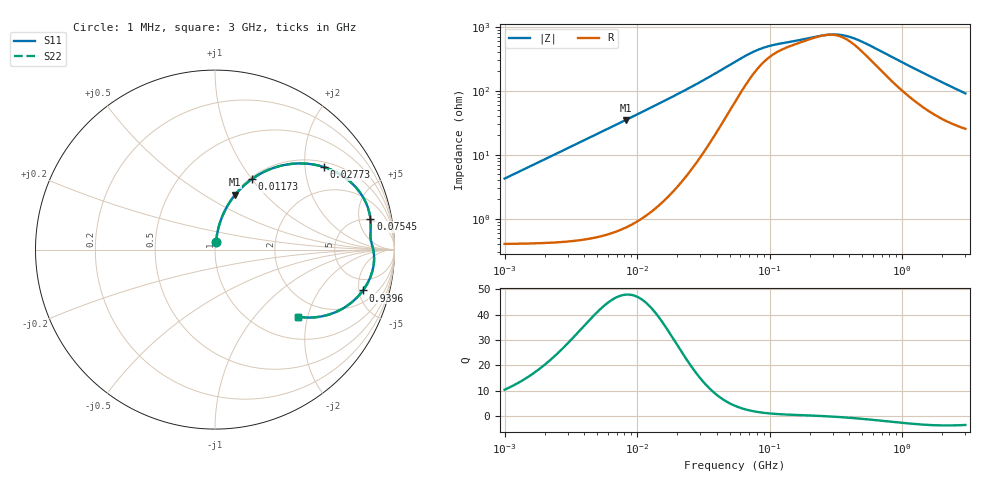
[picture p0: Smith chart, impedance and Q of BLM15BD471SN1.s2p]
! BLM15BD471SN1
# Hz S RI R 50
!Freq.(Hz) S11(Real) S11(Imag) S21(Real) S21(Imag) S12(Real) S12(Imag) S22(Real) S22(Imag)
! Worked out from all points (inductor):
!   401 points, 1 MHz to 3 GHz, reference 50 ohm
!   read as one part in series: L = 672 nH near 1.041 MHz
!   highest Q = 47.9 at 8.18 MHz (marker M1), where L = 676 nH
!   self-resonance near 267.3 MHz
!   S11 on the Smith chart (normalised r, x): 1 MHz: 1.01, +0.08; 11.73 MHz: 1.02, +1.00; 27.73 MHz: 1.15, +2.51; 75.45 MHz: 4.68, +7.24; 939.6 MHz: 3.25, -5.51; 3 GHz: 1.51, -1.74
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1000000  0.00579 0.0418  0.9942 -0.0418  0.9942 -0.0418  0.00579 0.0418
2055611  0.0116 0.0855  0.9884 -0.0855  0.9884 -0.0855  0.0116 0.0855
3823119  0.0298 0.1561  0.9702 -0.1561  0.9702 -0.1561  0.0298 0.1561
5820586  0.062 0.23  0.938 -0.23  0.938 -0.23  0.062 0.23
8179831  0.1129 0.3061  0.8871 -0.3061  0.8871 -0.3061  0.1129 0.3061
1.172775e7  0.2064 0.3937  0.7936 -0.3937  0.7936 -0.3937  0.2064 0.3937
1.461624e7  0.2889 0.4406  0.7111 -0.4406  0.7111 -0.4406  0.2889 0.4406
2.054061e7  0.4504 0.4795  0.5496 -0.4795  0.5496 -0.4795  0.4504 0.4795
2.773354e7  0.6056 0.4605  0.3944 -0.4605  0.3944 -0.4605  0.6056 0.4605
3.976269e7  0.7599 0.3722  0.2401 -0.3722  0.2401 -0.3722  0.7599 0.3722
5.477226e7  0.8388 0.2657  0.1612 -0.2657  0.1612 -0.2657  0.8388 0.2657
7.544761e7  0.866 0.1711  0.134 -0.1711  0.134 -0.1711  0.866 0.1711
1.060286e8  0.8668 0.1036  0.1332 -0.1036  0.1332 -0.1036  0.8668 0.1036
2.094008e8  0.8744 0.0283  0.1256 -0.0283  0.1256 -0.0283  0.8744 0.0283
2.884452e8  0.8833 -0.00987  0.1167 0.00987  0.1167 0.00987  0.8833 -0.00987
3.741707e8  0.8865 -0.0476  0.1135 0.0476  0.1135 0.0476  0.8865 -0.0476
4.853736e8  0.883 -0.0916  0.117 0.0916  0.117 0.0916  0.883 -0.0916
8.005644e8  0.847 -0.1922  0.153 0.1922  0.153 0.1922  0.847 -0.1922
9.395906e8  0.8243 -0.2277  0.1757 0.2277  0.1757 0.2277  0.8243 -0.2277
1.294266e9  0.7573 -0.2974  0.2427 0.2974  0.2427 0.2974  0.7573 -0.2974
1.818868e9  0.6525 -0.356  0.3475 0.356  0.3475 0.356  0.6525 -0.356
3e9  0.4625 -0.3736  0.5375 0.3736  0.5375 0.3736  0.4625 -0.3736
